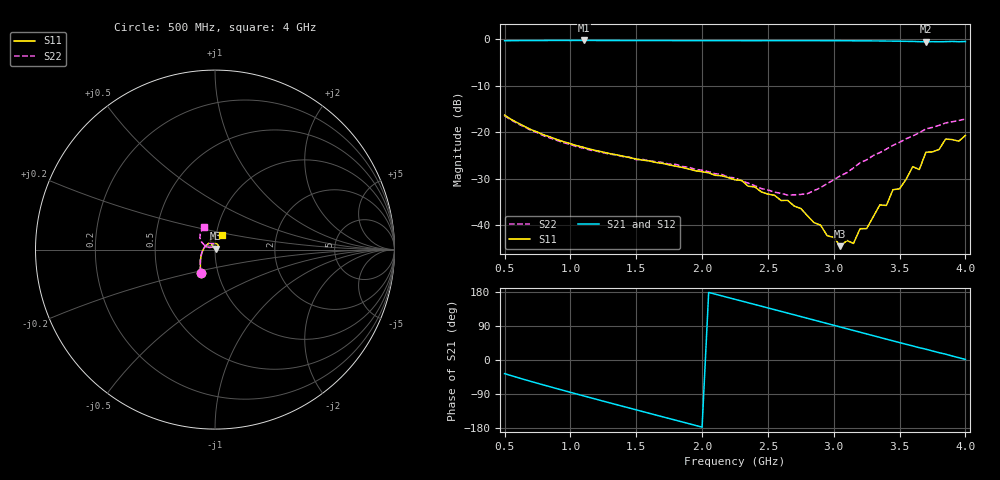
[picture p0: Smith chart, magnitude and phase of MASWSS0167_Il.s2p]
!Part No	MASWSS0167
!Fixture No	1000013396 REV B
! 2/8/2007  1:06:50 PM	Sample Board de-embdedding pS of delay  RFC 107.1	RF1 109.6
!EA:	CMS
!File Comment	AQTN 1888
!MASWSS0167_3V_4T_CMS.txt	MASWSS0167_4T_ testtitle_A
!Power Level	-5
!Test#	1	1	 Comments
!Fixture Loss is only removed from dB data
!measured state	RF to RF 1 IL
! Created Fri Feb 09 13:31:33 2007
!PORT 1= RFC  PORT2 = RF1
! Created Fri Feb 09 13:32:26 2007
# hz S db R 50
! 2 Port Network Data from SP1.SP block
! freq  dbS11  angS11  dbS21  angS21  dbS12  angS12  dbS22  angS22
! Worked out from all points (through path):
!   71 points, 500 MHz to 4 GHz, reference 50 ohm
!   highest |S21| = -0.24 dB at 1.1 GHz (marker M1); lowest = -0.5 dB at 3.7 GHz (marker M2)
!   group delay of S21, straight-line fit = 254 ps
!   lowest |S11| = -44.4 dB at 3.05 GHz (marker M3), VSWR 1.01, Z = 50.3 + j0.514 ohm
!   |S11| at or under -10 dB: start of sweep to end of sweep
!   |S22| runs from -33.5 to -16.4 dB; largest |S21 - S12| = 0.0012
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5e8  -16.30 -120.7  -0.31 -35.9  -0.31 -36.0  -16.44 -121.8
8e8  -20.55 -147.8  -0.25 -66.3  -0.26 -66.3  -20.76 -150.6
1.1e9  -23.22 -174.5  -0.24 -94.7  -0.25 -94.7  -23.39 -178.3
1.4e9  -25.11 156.4  -0.26 -122.4  -0.26 -122.4  -25.23 156.0
1.7e9  -26.67 123.8  -0.27 -149.9  -0.27 -149.9  -26.46 132.1
2e9  -28.44 91.0  -0.28 -177.2  -0.28 -177.2  -28.12 115.0
2.25e9  -30.19 61.4  -0.29 160.1  -0.29 160.1  -29.78 106.0
2.65e9  -34.61 30.3  -0.28 123.7  -0.28 123.7  -33.48 121.3
2.85e9  -39.40 23.8  -0.29 105.4  -0.29 105.4  -32.53 144.8
3.05e9  -44.45 58.5  -0.30 87.1  -0.31 87.1  -29.34 159.7
3.15e9  -43.86 90.1  -0.32 77.9  -0.32 77.9  -27.63 159.4
3.2e9  -40.69 105.2  -0.32 73.4  -0.32 73.3  -26.52 160.3
3.25e9  -40.68 104.8  -0.33 68.7  -0.34 68.7  -25.90 160.4
3.35e9  -35.58 112.8  -0.35 59.6  -0.35 59.6  -24.34 157.9
3.4e9  -35.70 127.3  -0.38 55.0  -0.38 55.0  -23.58 156.4
3.45e9  -32.31 124.6  -0.38 50.5  -0.38 50.5  -22.78 154.1
3.5e9  -32.13 120.0  -0.40 45.9  -0.41 45.9  -22.14 152.4
3.6e9  -27.36 116.8  -0.45 37.1  -0.45 37.1  -20.76 147.1
3.65e9  -27.99 120.8  -0.50 32.4  -0.50 32.4  -20.08 144.9
3.7e9  -24.26 116.5  -0.53 28.5  -0.53 28.5  -19.25 140.9
3.85e9  -21.43 91.3  -0.50 15.4  -0.50 15.3  -17.96 128.5
4e9  -20.66 64.4  -0.47 1.6  -0.47 1.5  -17.13 117.0
